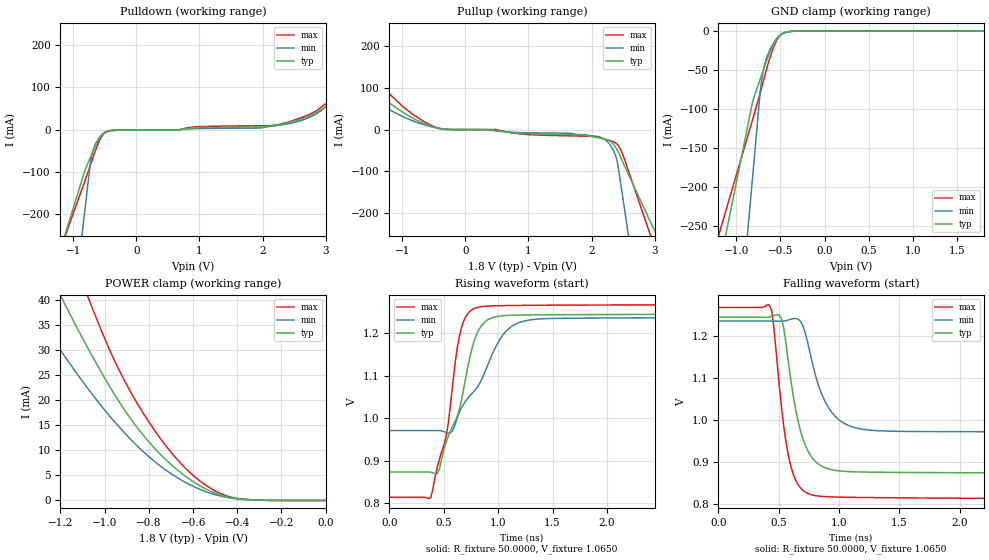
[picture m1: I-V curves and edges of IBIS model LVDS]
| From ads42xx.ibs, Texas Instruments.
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|   Model LVDS
[Model]  LVDS
Model_type 3-state
Polarity   Non-Inverting
Enable   Active-Low
Vmeas = 1.065V
Cref = 5.0000pF
Rref = 50.0000
Vref = 1.065V
C_comp   2.2000pF   2.0000pF   2.4000pF
[Temperature Range]   25.0000   0.1250k   -40.0000
[Voltage Range]   1.8000V   1.7000V   1.9000V
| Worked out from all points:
|   slope of the pulldown table from 0 to 0.27 V, typ, clamps not added: 2.09 kohm
|   slope of the pullup table from 0 to 0.27 V, typ, clamps not added: 19.8 kohm
|   GND clamp passes 1 mA (typ) near -0.42 V on its own axis
|   POWER clamp passes 1 mA (typ) near -0.47 V on its own axis
|   rising waveform, R_fixture 50.0000, V_fixture 1.0650: 20-80 % time 239ps typ, 353ps min, 171ps max; typ from 0.874 V to 1.25 V
|   falling waveform, R_fixture 50.0000, V_fixture 1.0650: 20-80 % time 145ps typ, 183ps min, 115ps max; typ from 1.25 V to 0.874 V
[Pulldown]
|Voltage   I(typ)   I(min)   I(max)
-1.8V     -573mA     -1.461A    -533.1mA
-810mV    -94.95mA   -186.3mA   -119.6mA
-730mV    -66.66mA   -83.27mA   -85.88mA
-680mV    -49.27mA   -46.93mA   -63.56mA
-570mV    -17.18mA   -16.04mA   -21.95mA
-460mV    -3.565mA   -3.744mA   -4.641mA
2.14V     8.453mA    8.285mA    9.976mA
2.69V     29.34mA    25.89mA    32.85mA
3.08V     59.8mA     67.4mA     70.71mA
3.15V     64.94mA    86.8mA     79.08mA
3.37V     96.85mA    188.2mA    102mA
3.6V      145.7mA    294.8mA    125.5mA
[Pullup]
|Voltage   I(typ)   I(min)   I(max)
-1.8V     134.2mA    249.1mA    177.6mA
-1.46V    93.73mA    90.29mA    125.5mA
-1.3V     74.94mA    57mA       101mA
-840mV    28.4mA     21.8mA     37.9mA
-400mV    2.545mA    3.108mA    2.645mA
1.67V     -11.52mA   -8.772mA   -14.8mA
2.17V     -20.9mA    -20.09mA   -21.51mA
2.3V      -27.99mA   -37.7mA    -26.34mA
2.39V     -44.22mA   -66.63mA   -32.8mA
2.43V     -55.47mA   -97.42mA   -39.42mA
2.52V     -86.2mA    -188.7mA   -70.02mA
3.6V      -438.5mA   -1.285A    -548.9mA
[GND_clamp]
|Voltage   I(typ)   I(min)   I(max)
-1.8V     -644.2mA   -1.444A    -493.9mA
-820mV    -93.96mA   -194.4mA   -115.6mA
-730mV    -62.28mA   -79.59mA   -80.23mA
-720mV    -58.98mA   -69.41mA   -75.99mA
-700mV    -52.31mA   -54.38mA   -67.41mA
-670mV    -42.41mA   -39.65mA   -54.64mA
-620mV    -27.2mA    -24.38mA   -34.87mA
-550mV    -11.15mA   -11.01mA   -13.8mA
-490mV    -3.867mA   -4.474mA   -4.534mA
-420mV    -941.3uA   -1.223mA   -1.169mA
-290mV    -42.52uA   -65.45uA   -73.57uA
1.8V      5.758nA    683.2nA    1.459nA
[POWER_clamp]
|Voltage   I(typ)   I(min)   I(max)
-1.8V     132.7mA    318.5mA    134.1mA
-1.32V    51.78mA    38.91mA    70.46mA
-1.26V    46.2mA     34.09mA    62.77mA
-1.18V    39.07mA    28.66mA    52.85mA
-1.07V    29.83mA    21.92mA    39.87mA
-940mV    20.04mA    14.91mA    26.44mA
-840mV    13.79mA    10.33mA    18.41mA
-730mV    8.407mA    6.259mA    11.26mA
-590mV    3.479mA    2.626mA    4.624mA
-490mV    1.299mA    1.039mA    1.675mA
-410mV    423.1uA    368.9uA    490.9uA
0V        5.758nA    60.92nA    1.932nA
[Ramp]
| variable   typ   min   max
dV/dt_r  0.6908/0.1782n   0.6769/0.2895n   0.6959/0.1276n
dV/dt_f  0.4915/0.2892n   0.4375/0.5015n   0.5288/0.1958n
R_load = 1.0000k
[Rising Waveform]
R_fixture= 50.0000
V_fixture= 1.0650
V_fixture_min= 1.1050
V_fixture_max= 1.0450
|time   V(typ)   V(min)   V(max)
0s        873.7mV    971.1mV    814.1mV
380ps     873.4mV    971.1mV    813mV
440ps     869.8mV    971.3mV    884.5mV
520ps     942.6mV    966.9mV    955.9mV
660ps     1.04V      1.024V     1.211V
780ps     1.183V     1.064V     1.258V
880ps     1.228V     1.11V      1.264V
1.1ns     1.242V     1.212V     1.265V
1.48ns    1.244V     1.235V     1.266V
20ns      1.245V     1.24V      1.267V
[Falling Waveform]
R_fixture= 50.0000
V_fixture= 1.0650
V_fixture_min= 1.1050
V_fixture_max= 1.0450
|time   V(typ)   V(min)   V(max)
0s        1.245V     1.236V     1.268V
420ps     1.245V     1.236V     1.274V
460ps     1.249V     1.236V     1.219V
520ps     1.244V     1.236V     1.037V
600ps     1.095V     1.24V      890.4mV
700ps     955.8mV    1.224V     832.9mV
860ps     889.9mV    1.059V     818.5mV
1.06ns    877.9mV    989.8mV    816.5mV
1.48ns    875.7mV    973.5mV    815.2mV
20ns      873.7mV    971.8mV    813.7mV
